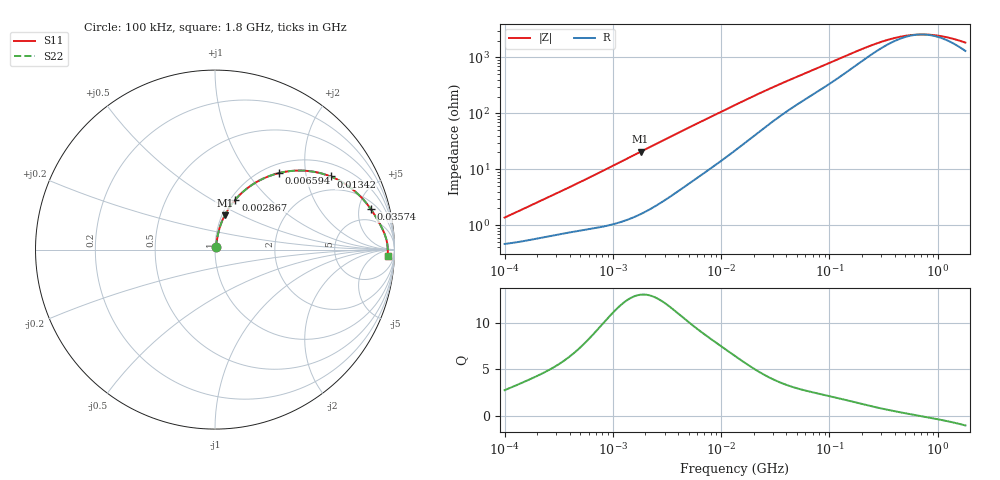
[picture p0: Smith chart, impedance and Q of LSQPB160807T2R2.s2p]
! LSQPB160807T2R2  S-PARAMETER MODEL  ( General Type )
! Model Generated by TAIYO YUDEN Corporation (http://www.ty-top.com)
! Version 1.0
! TAIYO YUDEN Control No. 110308NG25SB-FKC
! Copyright(c) 2011 TAIYO YUDEN CO.,LTD. All Rights Reserved.
! Product Description (link to TY-COMPAS)
! https://ds.yuden.co.jp/TYCOMPAS/or/detail?pn=LSQPB160807T2R2M&u=M
! Products Name : Inductors
! Characteristics :
!  Inductance : 2.2 uH , SRF(min) : 400 MHz , DC Resistance(max) : 0.52 Ohm
!  Rated Current : Saturation :360 mA , Temp Rise : 500 mA (40 degC)
!  Case Size : 1.6 x 0.8 / 0.063 x 0.031 [mm/inch] , Thickness : 0.7 / 0.028 [mm/inch]
!  (Conditions: Temperature = 25 degC , DC Bias Current/Voltage = 0A / 0V)
! External Node Assignments :
!  1  o---GGG---o  2
! GND o---------o GND
! Frequency Range : 0.1MHz  -  1800MHz  [ 402 STEP ]
# MHz S RI R 50
! Freq[MHz].  S11 Real  S11 Imag  S21 Real  S21 Imag  S12 Real  S12 Imag  S22 Real  S22 Imag
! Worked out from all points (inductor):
!   401 points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, 100 kHz to 1.8 GHz, reference 50 ohm
!   read as one part in series: L = 2.02 uH near 113 kHz
!   highest Q = 13 at 1.8 MHz (marker M1), where L = 1.81 uH
!   self-resonance near 704.6 MHz
!   S11 on the Smith chart (normalised r, x): 100 kHz: 1.01, +0.03; 2.867 MHz: 1.05, +0.65; 6.594 MHz: 1.16, +1.43; 13.42 MHz: 1.43, +2.78; 35.74 MHz: 2.84, +6.56; 1.8 GHz: 27, -26
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0.1  0.00477 0.0128  0.9952 -0.0128  0.9952 -0.0128  0.00477 0.0128
0.253659  0.00723 0.0306  0.9928 -0.0306  0.9928 -0.0306  0.00723 0.0306
0.516129  0.0116 0.0594  0.9884 -0.0594  0.9884 -0.0594  0.0116 0.0594
0.999975  0.0229 0.1112  0.9771 -0.1112  0.9771 -0.1112  0.0229 0.1112
1.800136  0.054 0.1907  0.946 -0.1907  0.946 -0.1907  0.054 0.1907
2.66389  0.1008 0.2638  0.8992 -0.2638  0.8992 -0.2638  0.1008 0.2638
2.867021  0.1133 0.2788  0.8867 -0.2788  0.8867 -0.2788  0.1133 0.2788
4.347904  0.211 0.3638  0.789 -0.3638  0.789 -0.3638  0.211 0.3638
6.593697  0.3565 0.4266  0.6435 -0.4266  0.6435 -0.4266  0.3565 0.4266
9.291023  0.4983 0.4396  0.5017 -0.4396  0.5017 -0.4396  0.4983 0.4396
13.41641  0.644 0.4075  0.356 -0.4075  0.356 -0.4075  0.644 0.4075
17.14029  0.7242 0.3664  0.2758 -0.3664  0.2758 -0.3664  0.7242 0.3664
21.36789  0.7814 0.3234  0.2186 -0.3234  0.2186 -0.3234  0.7814 0.3234
35.74074  0.8671 0.2272  0.1329 -0.2272  0.1329 -0.2272  0.8671 0.2272
69.24595  0.9214 0.1375  0.0786 -0.1375  0.0786 -0.1375  0.9214 0.1375
118.6955  0.9448 0.0869  0.0552 -0.0869  0.0552 -0.0869  0.9448 0.0869
213.6735  0.9569 0.0477  0.0431 -0.0477  0.0431 -0.0477  0.9569 0.0477
357.3983  0.961 0.0238  0.039 -0.0238  0.039 -0.0238  0.961 0.0238
528.8877  0.9622 0.0095  0.0378 -0.0095  0.0378 -0.0095  0.9622 0.0095
782.6622  0.9627 -0.00345  0.0373 0.00345  0.0373 0.00345  0.9627 -0.00345
1158.204  0.9625 -0.017  0.0375 0.017  0.0375 0.017  0.9625 -0.017
1800  0.9616 -0.0354  0.0384 0.0354  0.0384 0.0354  0.9616 -0.0354
